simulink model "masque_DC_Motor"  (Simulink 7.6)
settings: Solver=ode45  StartTime=0.0  StopTime=10.0  RelTol=1e-3
undefined symbols (not defined in the file or in its folder): Damp
libraries: fl_lib x8, nesl_utility x3

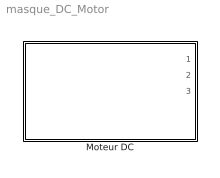
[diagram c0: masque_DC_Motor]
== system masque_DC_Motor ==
  Moteur DC : Subsystem  mask(Masque du moteur à courant continu avec des couples résistants appliqués à son arbre){R=0, L=0, K=0}
      mask prompts: R "Résistance d'induit, Ohm:"; L "Self d'induit, H:"; K "Paramètre électromécanique, V/(rad/s):"
      mask help: Masque du moteur à courant continu dont on spécifie : - la résistance d'induit, R (Ohm) - la self d'induit, L (Henry) - le paramètre électromécanique, K () reliant le couple moteur au courant d'induit On prévoit des couples résistants qu'on applique à son arbre : - Couple de frottement, fr en m N - Une inertie, J en g*cm^2 - Un amortissement, Damp en N*m/(rad/s)
      mask init:
      | clc
      | 
      | R=3.9;
      | L=12e-6;
      | K=0.072e-3*60/(2*pi);

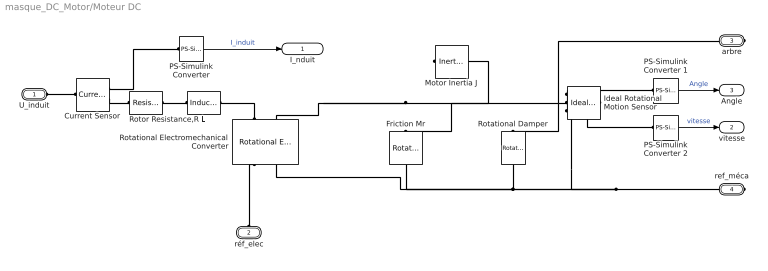
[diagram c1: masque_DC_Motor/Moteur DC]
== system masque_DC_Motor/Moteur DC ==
  Current Sensor : fl_lib/Electrical/Electrical Sensors/Current Sensor  DialogController=NetworkEngine.DynNeDlgSource  SystemSampleTime=-1  i1_Log=off  v1_Log=off  LocalVarNames=|i1|v1  LocalVarDescs=|i1|v1  LocalVarLogging=[0 0]
  Friction Mr : fl_lib/Mechanical/Rotational Elements/Rotational Friction  DialogController=NetworkEngine.DynNeDlgSource  SystemSampleTime=-1  brkwy_trq=fr N*m  Col_trq=fr N*m  visc_coef=0 N*m/(rad/s)  trans_coef=10 s/rad  vel_thr=0.1 rad/s  t_Log=off  w_Log=off  LocalVarNames=|friction_torque|rel_velocity|power  LocalVarDescs=|Friction torque (N*m)|Relative velocity (rad/s)|Power (W)  LocalVarLogging=[0 0 0]
  Ideal Rotational Motion Sensor : fl_lib/Mechanical/Mechanical Sensors/Ideal Rotational Motion Sensor  DialogController=NetworkEngine.DynNeDlgSource  SystemSampleTime=-1  offset=0 rad  w_Log=off  t_Log=off  phi_Log=off  LocalVarNames=|w|t|phi  LocalVarDescs=|w|t|phi  LocalVarLogging=[]
  L : fl_lib/Electrical/Electrical Elements/Inductor  DialogController=NetworkEngine.DynNeDlgSource  SystemSampleTime=-1  l=L H  i0=0 A  r=0 Ohm  g=1e-09 1/Ohm  i_Log=off  v_Log=off  i_L_Log=off  LocalVarNames=|current|voltage|power  LocalVarDescs=|Inductor current (A) |Voltage across inductor (V)|Power (W)  LocalVarLogging=[0 0 0]
  Motor Inertia J : fl_lib/Mechanical/Rotational Elements/Inertia  DialogController=NetworkEngine.DynNeDlgSource  SystemSampleTime=-1  inertia=J g*cm^2  initial_velocity=0 rad/s  t_Log=off  LocalVarNames=|torque|velocity  LocalVarDescs=|Inertia torque (N*m)|Inertia absolute velocity (rad/s)  LocalVarLogging=[0 0]
  PS-Simulink Converter : nesl_utility/PS-Simulink Converter  DialogController=NetworkEngine.DynNeUtilDlgSource  SystemSampleTime=-1  PhysicalDomain=network_engine_domain  LeftPortType=input  RightPortType=output  SubClassName=ps_output  Unit=1  AffineConversion=off
  PS-Simulink Converter 1 : nesl_utility/PS-Simulink Converter  DialogController=NetworkEngine.DynNeUtilDlgSource  SystemSampleTime=-1  PhysicalDomain=network_engine_domain  LeftPortType=input  RightPortType=output  SubClassName=ps_output  Unit=rad  AffineConversion=off
  PS-Simulink Converter 2 : nesl_utility/PS-Simulink Converter  DialogController=NetworkEngine.DynNeUtilDlgSource  SystemSampleTime=-1  PhysicalDomain=network_engine_domain  LeftPortType=input  RightPortType=output  SubClassName=ps_output  Unit=rpm  AffineConversion=off
  Rotational Electromechanical Converter : fl_lib/Electrical/Electrical Elements/Rotational Electromechanical Converter  DialogController=NetworkEngine.DynNeDlgSource  SystemSampleTime=-1  K=K V/(rad/s)  i_Log=off  v_Log=off  t_Log=off  w_Log=off  LocalVarNames=|current|voltage|power|torque|speed  LocalVarDescs=|Current (A)|Voltage (V)|Power (W)|Torque (Nm)|Angular speed (rad/s)  LocalVarLogging=[0 0 0 0 0]
  Rotational Damper : fl_lib/Mechanical/Rotational Elements/Rotational Damper  DialogController=NetworkEngine.DynNeDlgSource  SystemSampleTime=-1  D=Damp N*m/(rad/s)  t_Log=off  w_Log=off  LocalVarNames=|t|w  LocalVarDescs=|t|w  LocalVarLogging=[0 0]
  Rotor Resistance,R : fl_lib/Electrical/Electrical Elements/Resistor  Tag=Factory Generic  DialogController=NetworkEngine.DynNeDlgSource  SystemSampleTime=-1  R=R Ohm  i_Log=off  v_Log=off  LocalVarNames=|current|voltage|power  LocalVarDescs=|Resistor current (A)|Voltage across resistor (V)|Power (W)  LocalVarLogging=[0 0 0]
  U_induit : PMIOPort  Port=1  Side=Left
  réf_elec : PMIOPort  Port=2  Side=Left
  arbre : PMIOPort  Port=3  Side=Right
  ref_méca : PMIOPort  Port=4  Side=Right
  I_nduit : Outport
  vitesse : Outport  Port=2
  Angle : Outport  Port=3
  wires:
  PS-Simulink Converter 2/1 -> vitesse/1  "vitesse"
  PS-Simulink Converter 1/1 -> Angle/1  "Angle"
  PS-Simulink Converter/1 -> I_nduit/1  "I_induit"
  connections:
  réf_elec/RConn1 -- Rotational Electromechanical Converter/RConn1
  U_induit/RConn1 -- Current Sensor/LConn1
  Rotational Electromechanical Converter/LConn1 -- L/RConn1
  L/LConn1 -- Rotor Resistance,R/RConn1
  Ideal Rotational Motion Sensor/RConn3 -- PS-Simulink Converter 1/LConn1
  Ideal Rotational Motion Sensor/RConn2 -- PS-Simulink Converter 2/LConn1
  Ideal Rotational Motion Sensor/RConn1 -- Rotational Damper/RConn1 -- Rotational Electromechanical Converter/RConn2 -- Friction Mr/RConn1 -- ref_méca/RConn1
  Ideal Rotational Motion Sensor/LConn1 -- Rotational Damper/LConn1 -- Friction Mr/LConn1 -- Rotational Electromechanical Converter/LConn2 -- Motor Inertia J/LConn1 -- arbre/RConn1
  Current Sensor/RConn2 -- Rotor Resistance,R/LConn1
  Current Sensor/RConn1 -- PS-Simulink Converter/LConn1
